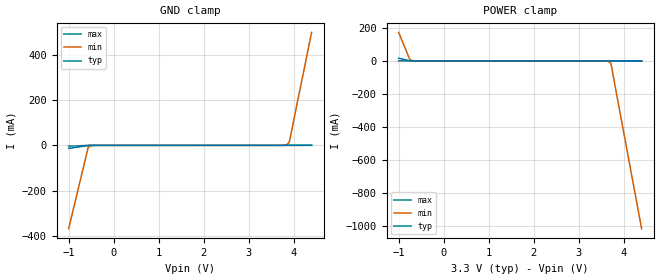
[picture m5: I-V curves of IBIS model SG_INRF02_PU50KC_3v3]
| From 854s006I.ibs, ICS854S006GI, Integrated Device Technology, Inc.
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[Model] SG_INRF02_PU50KC_3v3
Model_type   Input
Polarity   Non-Inverting
Vinl = 0.8V
Vinh = 2.0V
|   typ   min   max
C_comp   2pF   1.5pF   2.5pF
|   typ   min   max
[Voltage range]   3.3V   3.135V   3.465V
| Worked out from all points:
|   GND clamp passes 1 mA (typ) near -0.58 V on its own axis
|   POWER clamp passes 1 mA (typ) near -0.76 V on its own axis
[GND_clamp]
|Voltage   I (typ)   I (min)   I (max)
-999mV    -13.47mA   -368.7mA   -3.691mA
-564.6mV  -666.8uA   -8.599mA   -319.5uA
-502.5mV  -243.8uA   -1.423mA   -121.7uA
3.841V    13.44uA    2.09mA     6.981uA
3.904V    25.86uA    13.7mA     8.133uA
4.4V      415.2uA    499.8mA    17.43uA
[Power_clamp]
|Voltage   I (typ)   I (min)   I (max)
-999mV    16.01mA    172.7mA    690.8uA
-750.8mV  558.7uA    7.945mA    57.6uA
-688.7mV  119uA      1.251mA    21.36uA
3.531V    -69.78uA   -142.7uA   -65.48uA
3.655V    -74.91uA   -2.33mA    -67.78uA
3.717V    -92.13uA   -14.86mA   -68.93uA
4.4V      -989.7uA   -1.017A    -81.84uA
